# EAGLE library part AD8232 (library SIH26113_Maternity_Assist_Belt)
Analog Devices AD8232ACPZ-R7 single-lead heart-rate monitor front end. Supply 2.0-3.5 V. Pin map from AD8232 Rev.A Table 3.
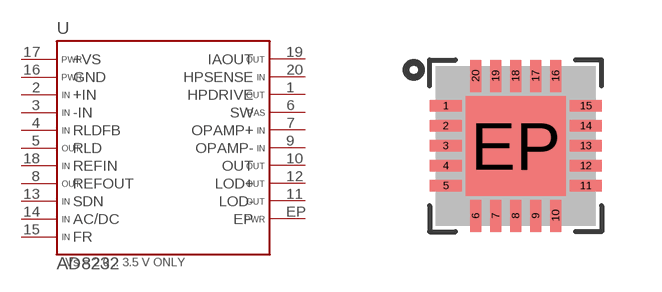
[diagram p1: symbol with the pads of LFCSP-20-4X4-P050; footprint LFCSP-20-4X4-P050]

Designator prefix U

## AD8232  [LFCSP-20-4X4-P050]
1  HPDRIVE  out
2  +IN  in
3  -IN  in
4  RLDFB  in
5  RLD  out
6  SW  pas
7  OPAMP+  in
8  REFOUT  out
9  OPAMP-  in
10  OUT  out
11  LOD-  out
12  LOD+  out
13  SDN  in
14  AC/DC  in
15  FR  in
16  GND  pwr
17  +VS  pwr
18  REFIN  in
19  IAOUT  out
20  HPSENSE  in
EP  EP  pwr

## Footprint LFCSP-20-4X4-P050 (pad centres in mm)
20-lead LFCSP_WQ 4x4 mm, 0.5 mm pitch, 2.50 mm SQ exposed pad (ADI CP-20-10 / JEDEC MO-220-WGGD). Body+terminal dims verified from the AD8232 Rev.A outline drawing; lands are IPC-7351B Nominal (0.80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
smd 0.8 x 0.28: 1 -1.75,1; 2 -1.75,0.5; 3 -1.75,0; 4 -1.75,-0.5; 5 -1.75,-1; 11 1.75,-1; 12 1.75,-0.5; 13 1.75,0; 14 1.75,0.5; 15 1.75,1
smd 0.28 x 0.8: 6 -1,-1.75; 7 -0.5,-1.75; 8 0,-1.75; 9 0.5,-1.75; 10 1,-1.75; 16 1,1.75; 17 0.5,1.75; 18 0,1.75; 19 -0.5,1.75; 20 -1,1.75
smd 2.5 x 2.5: EP 0,0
